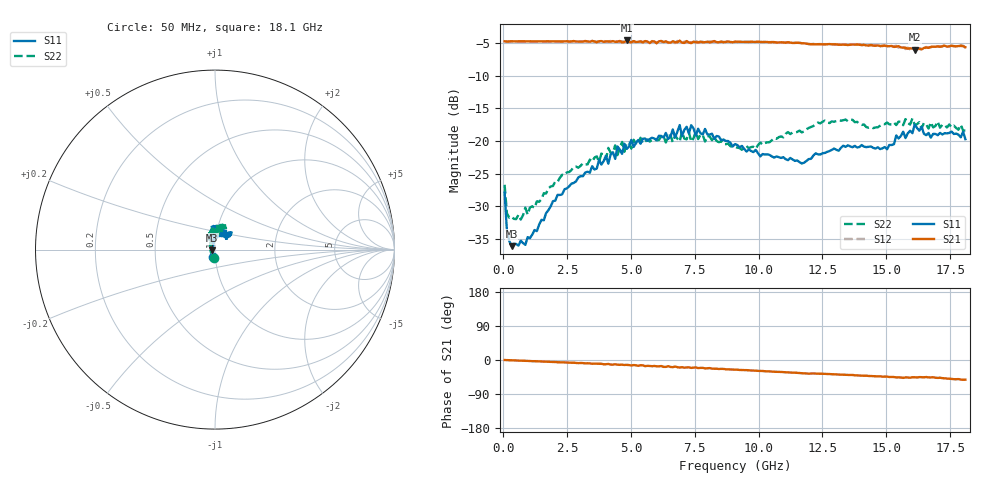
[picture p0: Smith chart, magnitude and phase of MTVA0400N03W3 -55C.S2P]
! Network Analyzer HP8720D.06.14 Serial No. US36140669
!  7 Jul 2005  13:31:04
! Frequency  S11  S21  S12  S22
# HZ  S  DB R 50
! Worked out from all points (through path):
!   201 points, 50 MHz to 18.1 GHz, reference 50 ohm
!   highest |S21| = -4.59 dB at 4.833 GHz (marker M1); lowest = -6.0 dB at 16.11 GHz (marker M2)
!   group delay of S21, straight-line fit = 8.1 ps
!   lowest |S11| = -36.1 dB at 320.8 MHz (marker M3), VSWR 1.03, Z = 48.5 - j0.439 ohm
!   |S11| at or under -10 dB: start of sweep to end of sweep
!   |S22| runs from -32.0 to -16.5 dB; largest |S21 - S12| = 0.021
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5e7  -27.90 -103.0  -4.72 -0.1  -4.72 0.2  -26.72 -95.6
1.4025e8  -33.77 -128.6  -4.77 -0.3  -4.75 -0.3  -31.08 -143.5
3.2075e8  -36.13 -163.2  -4.71 -0.7  -4.73 -0.7  -31.59 -170.6
6.8175e8  -35.30 164.8  -4.73 -1.7  -4.74 -1.7  -32.05 168.9
8.6225e8  -35.92 147.7  -4.73 -2.2  -4.74 -2.2  -30.23 161.6
9.525e8  -34.75 145.1  -4.73 -2.3  -4.73 -2.4  -31.29 154.4
2.12575e9  -28.27 101.9  -4.72 -5.9  -4.74 -5.8  -26.27 119.5
3.1185e9  -25.41 98.1  -4.76 -8.2  -4.78 -8.6  -23.42 118.2
4.83325e9  -21.22 94.6  -4.59 -12.8  -4.71 -13.9  -20.26 101.0
6.09675e9  -19.21 90.3  -4.72 -16.7  -4.66 -16.7  -19.85 100.3
6.7285e9  -19.47 95.0  -4.84 -17.2  -4.99 -18.2  -19.14 94.3
6.909e9  -17.57 93.7  -4.63 -19.9  -4.77 -19.0  -20.08 92.2
6.99925e9  -19.23 92.7  -4.92 -19.1  -4.95 -20.5  -18.56 93.7
7.36025e9  -17.58 87.5  -5.01 -20.9  -4.86 -19.9  -20.10 98.0
7.54075e9  -19.16 88.7  -4.86 -19.6  -4.71 -21.4  -18.58 98.0
7.90175e9  -18.16 96.1  -4.86 -22.3  -4.84 -21.4  -20.10 92.4
9.075e9  -20.48 103.8  -4.79 -25.4  -4.78 -25.4  -20.91 86.8
1.169225e10  -23.46 80.4  -5.02 -34.9  -5.01 -34.8  -18.68 73.4
1.21435e10  -22.25 77.9  -5.16 -35.5  -5.12 -35.7  -17.71 75.1
1.512175e10  -20.61 44.5  -5.47 -44.9  -5.33 -44.6  -17.46 74.3
1.61145e10  -17.48 45.9  -6.00 -45.6  -5.76 -45.8  -17.54 69.3
1.81e10  -19.72 65.8  -5.63 -51.9  -5.74 -52.8  -18.41 79.9
